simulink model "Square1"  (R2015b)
settings: Solver=VariableStepAuto  StartTime=0.0  StopTime=10.0  RelTol=1e-3
libraries: vexarmcortexlib x4

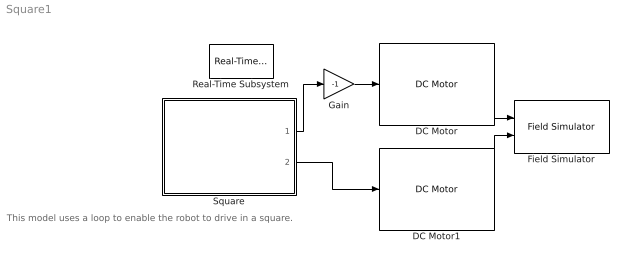
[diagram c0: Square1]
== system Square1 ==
  note: This model uses a loop to enable the robot to drive in a square.
  DC Motor : vexarmcortexlib/DC Motor  motor=3  scaleFactor=1/13.5  SimulationOut=on
  DC Motor1 : vexarmcortexlib/DC Motor  motor=7  scaleFactor=1/13.5  SimulationOut=on
  Field Simulator : vexarmcortexlib/Utilities/Field Simulator  radius=2.5  space=10  range=200
  Gain : Gain  Gain=-1
  Real-Time Subsystem : vexarmcortexlib/Utilities/Real-Time Subsystem  x=1
  Square : Stateflow chart  TreatAsAtomicUnit=on
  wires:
  DC Motor/1 -> Field Simulator/1
  DC Motor1/1 -> Field Simulator/2
  Gain/1 -> DC Motor/1
  Square/1(speedL) -> Gain/1
  Square/2(speedR) -> DC Motor1/1

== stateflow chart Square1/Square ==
  state Halt
    during:
    speedL = 0;
    speedR = 0;
  state TurnRight
    during:
    speedL = 42;
    speedR = -42;
  state Forward
    during:
    speedL = 100;
    speedR = 100;
    entry:
    count = count +1;
  state FullStop
    during:
    speedL = 0;
    speedR = 0;
  state Note that there is a counter which [group]
    increases the index every time the
    loop enters the State called Forward
  TurnRight -> Halt : after(1,sec)
  Halt -> Forward : after(1,sec)
  Forward -> TurnRight : after(4,sec)
  Forward -> FullStop : [count>4]
  (default) -> Forward : {count = 0;}
  data: speedL output; speedR output; count local
